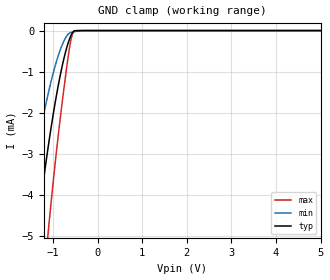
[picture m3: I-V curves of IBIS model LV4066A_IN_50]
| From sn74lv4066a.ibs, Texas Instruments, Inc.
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[Model]   LV4066A_IN_50
Model_type  Input
Vinl = 1.35
Vinh = 3.85
| variable   typ   min   max
C_comp   1.27pF   0.81pF   1.44pF
[Temperature Range]   40   100   -40
| Ambient temperature   25   85   -40
[Voltage range]   5   4.5   5.5
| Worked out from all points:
|   GND clamp passes 1 mA (typ) near -0.82 V on its own axis
[GND Clamp]
| LV4066A_IN_50
|   Voltage   I(typ)   I(min)   I(max)
-5V       -50.6mA    -35.31mA   -73.31mA
-1.695V   -8.057mA   -5.057mA   -12.66mA
-1.64V    -7.507mA   -4.678mA   -11.86mA
-1.35V    -4.799mA   -2.834mA   -7.873mA
-1.11V    -2.855mA   -1.552mA   -4.946mA
-975mV    -1.913mA   -958.1uA   -3.482mA
-835mV    -1.08mA    -466.9uA   -2.123mA
-710mV    -490.5uA   -165.2uA   -1.044mA
-610mV    -154.3uA   -49.56uA   -303.2uA
-555mV    -40.93uA   -34.18uA   -66.31uA
-510mV    -6.292uA   -25.2uA    -1.454uA
5V        20.25pA    158.4pA    15.01pA
